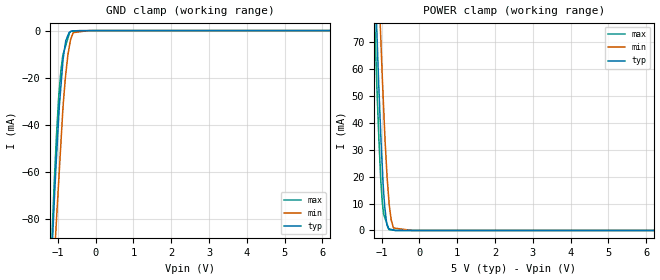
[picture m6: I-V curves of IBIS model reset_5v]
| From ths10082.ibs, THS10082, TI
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|   reset_5v Model
[Model]   reset_5v
Model_type   Input
Vinl = 0.6
Vinh = 2.6
|   typ   min   max
C_comp   9.413e-13   9.377e-13   9.450e-13
[Voltage Range]   5   4.75   5.25
|Ambient Temperature   25   85   -40
|Junction Temperature
[Temperature Range]   27   125   -40
[Power Clamp Reference]   5   4.75   5.25
[GND Clamp Reference]   0   0   0
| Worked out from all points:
|   GND clamp passes 1 mA (typ) near -0.71 V on its own axis
|   POWER clamp passes 1 mA (typ) near -0.83 V on its own axis
[GND Clamp]
|   Voltage   I(typ)   I(min)   I(max)
-5V       -1.717A    -1.634A    -1.818A
-1.306V   -147.3mA   -167.9mA   -146.6mA
-1.103V   -75.38mA   -100.7mA   -67.09mA
-1.08V    -67.57mA   -93.54mA   -59.35mA
-1.045V   -56.34mA   -82.68mA   -47.49mA
-976.5mV  -36.57mA   -63.68mA   -28.13mA
-865mV    -12.8mA    -32.95mA   -10.23mA
-790mV    -4.331mA   -18.47mA   -6.243mA
-736.2mV  -2.163mA   -10.64mA   -3.387mA
-640mV    -213.9uA   -2.839mA   -238.5uA
-190mV    0A         -23.42nA   -70.81uA
10V       0A         0A         0A
[POWER Clamp]
|   Voltage   I(typ)   I(min)   I(max)
-5V       1.838A     1.841A     1.848A
-1.306V   146.9mA    183.3mA    128.9mA
-1.129V   75.46mA    112.3mA    55.12mA
-1.024V   36.37mA    72.35mA    19.39mA
-981.8mV  23.69mA    57.19mA    10.52mA
-915mV    8.506mA    35.67mA    4.771mA
-860mV    2.278mA    21.24mA    2.606mA
-798mV    583.6uA    9.619mA    291.7uA
-745.8mV  395.6uA    3.899mA    204.9uA
-684mV    173.5uA    927.7uA    102.2uA
-190mV    0A         0A         8.884uA
10V       0A         0A         0A
